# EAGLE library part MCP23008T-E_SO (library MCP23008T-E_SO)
Interface - I/O Expanders In/Out I2C int Source: Datasheet
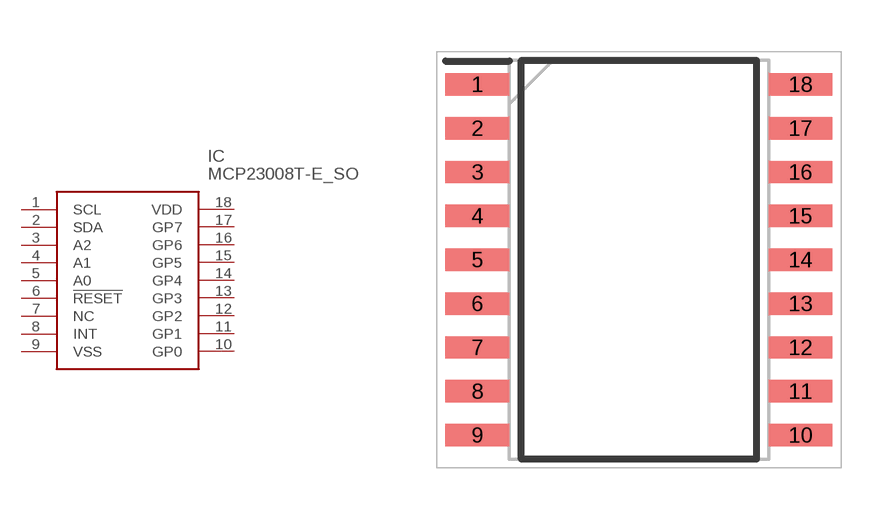
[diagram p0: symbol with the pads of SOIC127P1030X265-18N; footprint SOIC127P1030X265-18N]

Designator prefix IC

## MCP23008T-E_SO (Description: Interface - I/O Expanders In/Out I2C int; Height: 2.65mm; Manufacturer_Name: Microchip; Manufacturer_Part_Number: MCP23008T-E/SO; Mouser_Part_Number: 579-MCP23008T-E/SO; Mouser_Price-Stock: https://www.mouser.co.uk/ProductDetail/Microchip-Technology/MCP23008T-E-SO?qs=L9Ynyw3fbhGdT1w2KdF%2FLQ%3D%3D)  [SOIC127P1030X265-18N]
1  SCL
2  SDA
3  A2
4  A1
5  A0
6  !RESET
7  NC  nc
8  INT
9  VSS
10  GP0
11  GP1
12  GP2
13  GP3
14  GP4
15  GP5
16  GP6
17  GP7
18  VDD

## Footprint SOIC127P1030X265-18N (pad centres in mm)
DSPIC33FJ12GP201-I/SO-1
smd 1.85 x 0.65: 1 -4.675,5.08; 2 -4.675,3.81; 3 -4.675,2.54; 4 -4.675,1.27; 5 -4.675,0; 6 -4.675,-1.27; 7 -4.675,-2.54; 8 -4.675,-3.81; 9 -4.675,-5.08; 10 4.675,-5.08; 11 4.675,-3.81; 12 4.675,-2.54; 13 4.675,-1.27; 14 4.675,0; 15 4.675,1.27; 16 4.675,2.54; 17 4.675,3.81; 18 4.675,5.08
